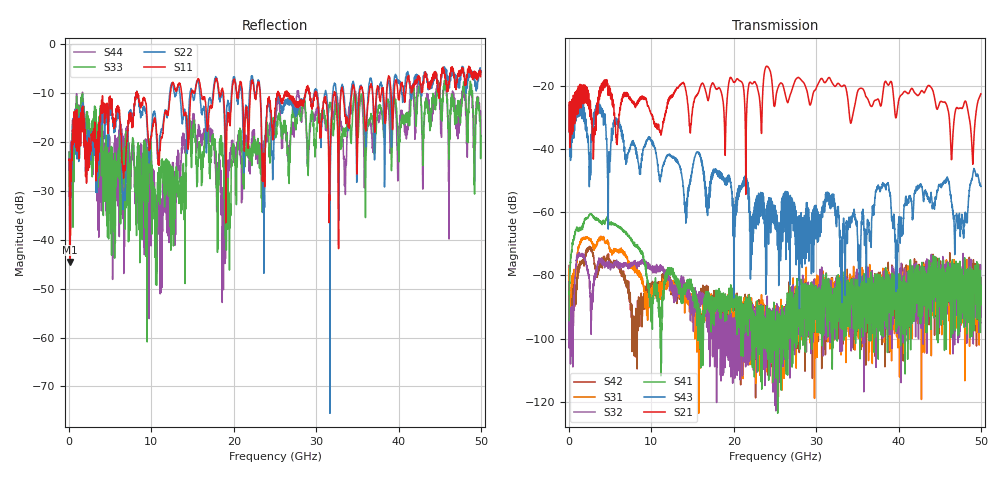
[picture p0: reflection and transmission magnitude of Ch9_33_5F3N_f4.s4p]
!Agilent Technologies,N5247A,US51170199,A.09.90.13
!Agilent N5247A: A.09.90.13
!Date: Wednesday, December 16, 2015 12:05:34
!Correction: S11(Full 4 Port(1,2,3,4))
!S12(Full 4 Port(1,2,3,4))
!S13(Full 4 Port(1,2,3,4))
!S14(Full 4 Port(1,2,3,4))
!S21(Full 4 Port(1,2,3,4))
!S22(Full 4 Port(1,2,3,4))
!S23(Full 4 Port(1,2,3,4))
!S24(Full 4 Port(1,2,3,4))
!S31(Full 4 Port(1,2,3,4))
!S32(Full 4 Port(1,2,3,4))
!S33(Full 4 Port(1,2,3,4))
!S34(Full 4 Port(1,2,3,4))
!S41(Full 4 Port(1,2,3,4))
!S42(Full 4 Port(1,2,3,4))
!S43(Full 4 Port(1,2,3,4))
!S44(Full 4 Port(1,2,3,4))
!S4P File: Measurements: <S11,S12,S13,S14>,
!<S21,S22,S23,S24>,
!<S31,S32,S33,S34>,
!<S41,S42,S43,S44>:
# Hz S  dB  R 50
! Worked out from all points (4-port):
!   3201 points, 10 MHz to 50 GHz, reference 50 ohm
!   strongest paths, dB at 10 MHz, 12.51 GHz, 25 GHz, 37.5 GHz, 50 GHz:
!     S21: -34.5, -23.5, -26.1, -24.2, -22.5
!     S43: -34.7, -42.7, -58.0, -52.0, -51.8
!     S41: -94.3, -78.1, -100.5, -89.4, -83.2
!     S32: -82.0, -85.2, -100.3, -81.2, -95.0
!     S31: -78.1, -83.9, -99.4, -100.9, -93.2
!     S42: -76.9, -82.9, -95.2, -102.5, -83.4
!   lowest |S11| = -44.5 dB at 88.11 MHz (marker M1), VSWR 1.01, Z = 50.4 + j0.482 ohm
!   |S11| at or under -10 dB: start of sweep to 8.126 GHz; 8.252 GHz to 12.29 GHz (4.042 GHz wide, 39.3 % of centre); 23.21 GHz to 25.35 GHz (2.141 GHz wide, 8.82 % of centre)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
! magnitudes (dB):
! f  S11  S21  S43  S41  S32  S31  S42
! 10 MHz  -23.8  -34.5  -34.7  -94.3  -82.0  -78.1  -76.9
! 88.11 MHz  -44.5  -39.6  -42.3  -81.8  -100.0  -89.0  -90.7
! 11.2 GHz  -19.1  -35.3  -48.6  -100.6  -76.9  -86.1  -83.2
! 15.09 GHz  -9.9  -26.0  -44.9  -85.0  -90.5  -94.9  -92.4
! 18.83 GHz  -12.1  -29.8  -49.4  -90.6  -94.8  -89.6  -94.2
! 35.24 GHz  -10.5  -21.0  -77.0  -82.3  -91.1  -83.9  -97.7
! 50 GHz  -5.6  -22.5  -51.8  -83.2  -95.0  -93.2  -83.4
